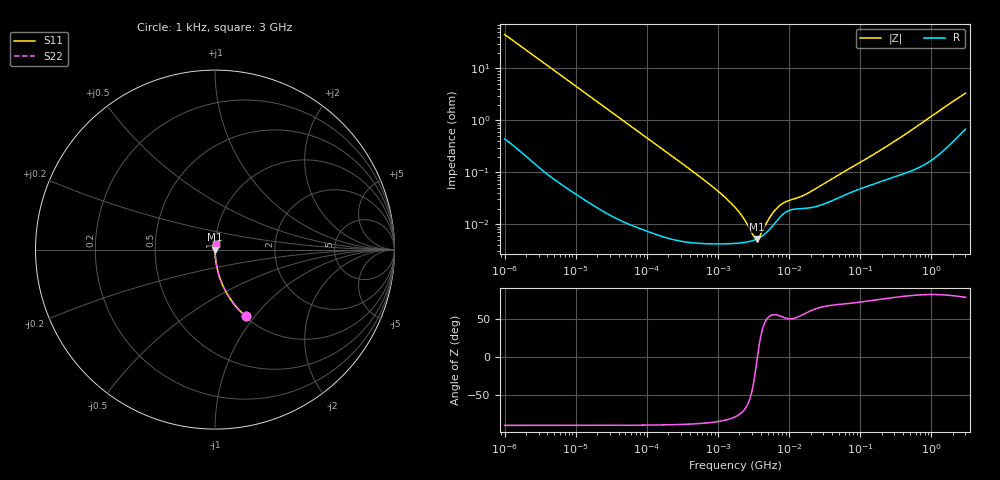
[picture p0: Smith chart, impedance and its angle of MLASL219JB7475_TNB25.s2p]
! MLASL219JB7475_TNB25  S-PARAMETER MODEL  ( Standard Model )
! Model Generated by TAIYO YUDEN Corporation (http://www.ty-top.com)
! Version 1.0
! TAIYO YUDEN Control No. 220601
! Copyright(c) 2010 TAIYO YUDEN CO.,LTD. All Rights Reserved.
! Product Description (link to TY-COMPAS)
! https://ds.yuden.co.jp/TYCOMPAS/or/detail?pn=MLASL219JB7475KTNB25&u=M
! Products Name : Multilayer Ceramic Capacitors
! Characteristics :
!  Capacitance : 4.7 [uF] , Rated Voltage : 10 [V] , TCC : X7R
!  Case Size : 2.0 x 1.25 / 0.079 x 0.049 [mm/inch] , Thickness : 0.85 / 0.033 [mm/inch]
!  (Conditions: Temperature = 25 [degC] , DC Bias Voltage = 0 [V])
! External Node Assignments :
!  1  o---| |---o  2
! GND o---------o GND
! Frequency Range : 1kHz  -  3GHz  [ 401 STEP ]
# MHZ S RI R 50
! Freq[MHz].  S11 Real  S11 Imag  S21 Real  S21 Imag  S12 Real  S12 Imag  S22 Real  S22 Imag
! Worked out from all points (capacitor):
!   401 points, 1 kHz to 3 GHz, reference 50 ohm
!   read as one part in series: C = 3.51 uF near 1.077 kHz
!   lowest |Z| = 5.22 mohm at 3.517 MHz (marker M1)
!   series resonance near 3.58 MHz, so ESL is about 560 pH
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0.001  0.1722 -0.3727  0.8278 0.3727  0.8278 0.3727  0.1722 -0.3727
0.001749  0.0651 -0.2421  0.9349 0.2421  0.9349 0.2421  0.0651 -0.2421
0.003297  0.0198 -0.1353  0.9802 0.1353  0.9802 0.1353  0.0198 -0.1353
0.005988  0.00639 -0.0758  0.9936 0.0758  0.9936 0.0758  0.00639 -0.0758
0.01216  0.00174 -0.0376  0.9983 0.0376  0.9983 0.0376  0.00174 -0.0376
0.147855  7.05e-05 -0.00313  0.9999 0.00313  0.9999 0.00313  7.05e-05 -0.00313
0.791611  4.22e-05 -0.000561  1 0.000561  1 0.000561  4.22e-05 -0.000561
1.238299  4.2e-05 -0.000333  1 0.000333  1 0.000333  4.2e-05 -0.000333
1.732051  4.27e-05 -0.000208  1 0.000208  1 0.000208  4.27e-05 -0.000208
2.422679  4.49e-05 -0.000106  1 0.000106  1 0.000106  4.49e-05 -0.000106
2.610246  4.57e-05 -8.54e-05  1 8.54e-05  1 8.54e-05  4.57e-05 -8.54e-05
2.812335  4.68e-05 -6.49e-05  1 6.49e-05  1 6.49e-05  4.68e-05 -6.49e-05
3.517417  5.2e-05 -4.71e-06  0.9999 4.71e-06  0.9999 4.71e-06  5.2e-05 -4.71e-06
4.566395  6.53e-05 6.63e-05  0.9999 -6.63e-05  0.9999 -6.63e-05  6.53e-05 6.63e-05
4.919932  7.16e-05 8.69e-05  0.9999 -8.69e-05  0.9999 -8.69e-05  7.16e-05 8.69e-05
6.387174  0.000107 0.000156  0.9999 -0.000156  0.9999 -0.000156  0.000107 0.000156
8.291982  0.000158 0.000202  0.9998 -0.000202  0.9998 -0.000202  0.000158 0.000202
15.05716  0.0002 0.000285  0.9998 -0.000285  0.9998 -0.000285  0.0002 0.000285
21.06097  0.000211 0.000387  0.9998 -0.000387  0.9998 -0.000387  0.000211 0.000387
256.0921  0.000765 0.00333  0.9992 -0.00333  0.9992 -0.00333  0.000765 0.00333
2066.299  0.00459 0.0233  0.9954 -0.0233  0.9954 -0.0233  0.00459 0.0233
3000  0.00776 0.0322  0.9922 -0.0322  0.9922 -0.0322  0.00776 0.0322
